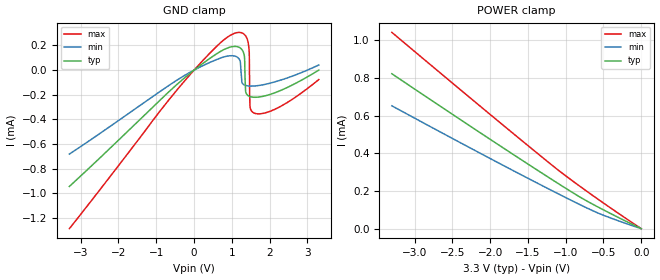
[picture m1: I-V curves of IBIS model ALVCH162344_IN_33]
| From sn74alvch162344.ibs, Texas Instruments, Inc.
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[Model]   ALVCH162344_IN_33
Model_type  Input
Vinl = 0.8
Vinh = 2.0
| variable   typ   min   max
C_comp   2.16pF   1.65pF   2.62pF
[Temperature Range]   40   100   -40
| Ambient temperature   25   85   -40
[Voltage range]   3.3   3   3.6
[GND Clamp]
| ALVCH162344_IN_33
|   Voltage   I(typ)   I(min)   I(max)
-3.3V     -943.7uA   -681.3uA   -1.286mA
950mV     186.1uA    116.2uA    280.5uA
1.205V    182.7uA    82.93uA    305.7uA
1.305V    144.3uA    -116uA     295.5uA
1.335V    104.4uA    -121.2uA   287.9uA
1.365V    -174.6uA   -124.5uA   276.8uA
1.415V    -203.5uA   -127.8uA   243.2uA
1.46V     -212.2uA   -129.3uA   143.5uA
1.47V     -213.5uA   -129.5uA   -174.9uA
1.48V     -214.6uA   -129.6uA   -295.1uA
1.58V     -220.2uA   -129.2uA   -347.2uA
3.3V      8.374pA    41.32uA    -77.01uA
[POWER Clamp]
| ALVCH162344_IN_33
|   Voltage   I(typ)   I(min)   I(max)
-3.3V     822.6uA    652.4uA    1.042mA
-2.08V    495.8uA    389.6uA    633.2uA
-1.105V   241.1uA    186.3uA    312.9uA
-800mV    165.2uA    125.3uA    221.5uA
-560mV    112.3uA    80.92uA    152.8uA
-48.03fV  8.374pA    8.764pA    8.53pA
